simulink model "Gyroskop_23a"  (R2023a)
settings: Solver=ode1  StartTime=0.0  StopTime=inf  FixedStep=0.0005  RelTol=1e-3  EnableMultiTasking=on
undefined symbols (not defined in the file or in its folder): dps, Hz
libraries: arduinosensorlib x1, dspindex x1

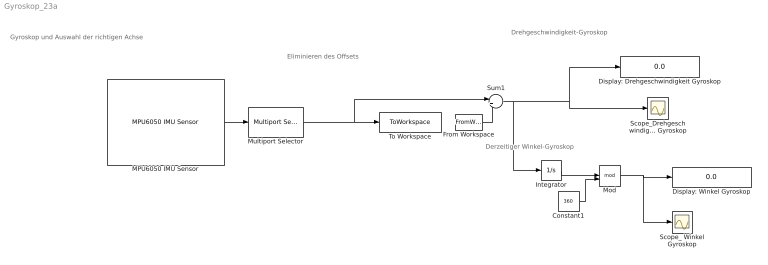
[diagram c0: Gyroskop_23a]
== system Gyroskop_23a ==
  note: Derzeitiger Winkel-Gyroskop
  note: Gyroskop und Auswahl der richtigen Achse
  note: Eliminieren des Offsets
  note: Drehgeschwindigkeit-Gyroskop
  Constant1 : Constant  Value=360
  Display: Drehgeschwindigkeit Gyroskop : Display
  Display: Winkel Gyroskop : Display
  From Workspace : FromWorkspace  VariableName=T
  Integrator : Integrator
  MPU6050 IMU Sensor : arduinosensorlib/MPU6050 IMU Sensor  SlaveAddress=0x68  Accel=off  AngularRate=on  Temperature=off  Status=off  Timestamp=off  EulerAngles=off  Quat=off  AccelRange=2G  GyroRange=250 dps  DmpOdr=200 Hz  Dlpf=Accelerometer: 184Hz, Gyroscope: 188Hz  spf=1  SampleTime=-1  QueueSizeFactor=1
  Mod : Math  Operator=mod
  Multiport Selector : dspindex/Multiport Selector  rowsOrCols=Rows  idxCellArray={1}  idxErrMode=Clip Index
  Scope_ Winkel Gyroskop : Scope
  Scope_Drehgeschwindigkeit Gyroskop : Scope
  Sum1 : Sum  Inputs=|+-
  To Workspace : ToWorkspace  VariableName=simout  SampleTime=-1
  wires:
  From Workspace/1 -> Sum1/2
  Multiport Selector/1 -> Sum1/1, To Workspace/1
  Constant1/1 -> Mod/2
  MPU6050 IMU Sensor/1 -> Multiport Selector/1
  Sum1/1 -> Scope_Drehgeschwindigkeit Gyroskop/1, Display: Drehgeschwindigkeit Gyroskop/1, Integrator/1
  Integrator/1 -> Mod/1
  Mod/1 -> Scope_ Winkel Gyroskop/1, Display: Winkel Gyroskop/1
